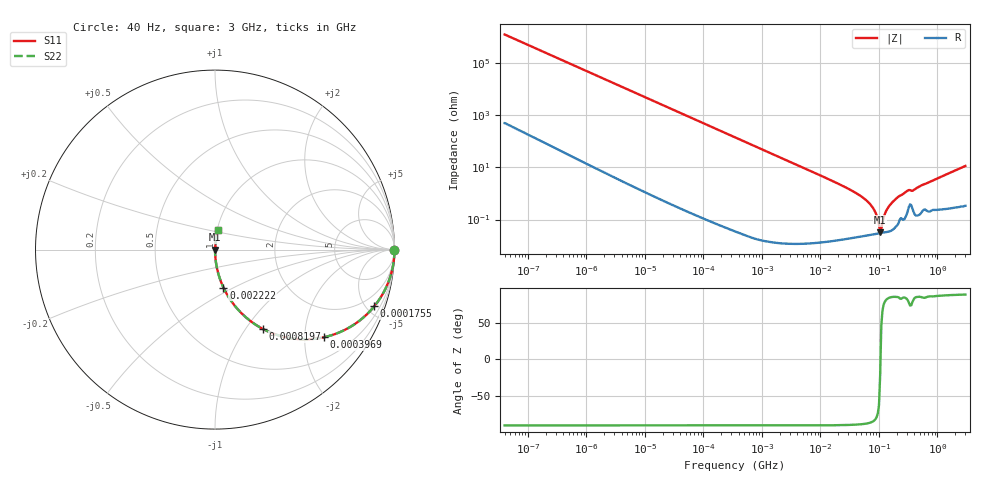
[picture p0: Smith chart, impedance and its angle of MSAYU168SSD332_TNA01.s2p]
! MSAYU168SSD332_TNA01  S-PARAMETER MODEL  ( General Type )
! Model Generated by TAIYO YUDEN Corporation (http://www.ty-top.com)
! Version 2.0
! TAIYO YUDEN Control No. 030711
! Copyright(c) 2003 TAIYO YUDEN CO.,LTD. All Rights Reserved.
! Product Description (link to TY-COMPAS)
! https://ds.yuden.co.jp/TYCOMPAS/or/detail?pn=MSAYU168SSD332KTNA01&u=M
! Products Name : Multilayer Ceramic Capacitors
! Characteristics :
!  Capacitance : 3300 pF , Rated Voltage : 50V
!  Case Size : 1.6 x 0.8 / 0.063 x 0.031 [mm/inch] , Thickness : 0.8 / 0.031 [mm/inch]
!  (Conditions: Temperature = 25 degC , DC Bias Current/Voltage = 0A / 0V)
! External Node Assignments :
!  1  o---| |---o  2
! GND o---------o GND
! Frequency Range : 40Hz  -  3GHz  [ 401 STEP ]
# MHz S RI R 50
! Freq[MHz].  S11 Real  S11 Imag  S21 Real  S21 Imag  S12 Real  S12 Imag  S22 Real  S22 Imag
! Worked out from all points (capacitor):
!   401 points, 40 Hz to 3 GHz, reference 50 ohm
!   read as one part in series: C = 3.23 nF near 44 Hz
!   lowest |Z| = 32.5 mohm at 104.8 MHz (marker M1)
!   series resonance near 106.1 MHz, so ESL is about 700 pH
!   S11 on the Smith chart (normalised r, x): 40 Hz: open; 175.5 kHz: 1.00, -5.62; 396.9 kHz: 1.00, -2.48; 819.7 kHz: 1.00, -1.20; 2.222 MHz: 1.00, -0.44; 3 GHz: 1.01, +0.23
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4e-05  1 -8.12e-05  3.9e-08 8.12e-05  3.9e-08 8.12e-05  1 -8.12e-05
5.3e-05  1 -0.000108  5.4e-08 0.000108  5.4e-08 0.000108  1 -0.000108
0.000834  1 -0.00169  3.35e-06 0.00169  3.35e-06 0.00169  1 -0.00169
0.017386  0.9987 -0.0352  0.00125 0.0352  0.00125 0.0352  0.9987 -0.0352
0.061867  0.9845 -0.1236  0.0155 0.1236  0.0155 0.1236  0.9845 -0.1236
0.175499  0.8874 -0.316  0.1126 0.316  0.1126 0.316  0.8874 -0.316
0.362475  0.6489 -0.4772  0.3511 0.4772  0.3511 0.4772  0.6489 -0.4772
0.396875  0.6066 -0.4884  0.3934 0.4884  0.3934 0.4884  0.6066 -0.4884
0.819702  0.2655 -0.4415  0.7345 0.4415  0.7345 0.4415  0.2655 -0.4415
2.222206  0.0469 -0.2112  0.9531 0.2112  0.9531 0.2112  0.0469 -0.2112
7.222098  0.00471 -0.0676  0.9953 0.0676  0.9953 0.0676  0.00471 -0.0676
28.13798  0.000445 -0.0163  0.9996 0.0163  0.9996 0.0163  0.000445 -0.0163
55.54024  0.000275 -0.00643  0.9997 0.00643  0.9997 0.00643  0.000275 -0.00643
79.8195  0.000275 -0.00268  0.9997 0.00268  0.9997 0.00268  0.000275 -0.00268
104.7695  0.000301 -0.000121  0.9997 0.000121  0.9997 0.000121  0.000301 -0.000121
114.7124  0.000313 0.000706  0.9997 -0.000706  0.9997 -0.000706  0.000313 0.000706
131.4235  0.000333 0.00202  0.9997 -0.00202  0.9997 -0.00202  0.000333 0.00202
150.5692  0.000362 0.00337  0.9996 -0.00337  0.9996 -0.00337  0.000362 0.00337
206.7996  0.000666 0.00696  0.9993 -0.00696  0.9993 -0.00696  0.000666 0.00696
297.2015  0.0017 0.0119  0.9983 -0.0119  0.9983 -0.0119  0.0017 0.0119
390.1008  0.00216 0.0132  0.9978 -0.0132  0.9978 -0.0132  0.00216 0.0132
3000  0.0159 0.1109  0.9841 -0.1109  0.9841 -0.1109  0.0159 0.1109
